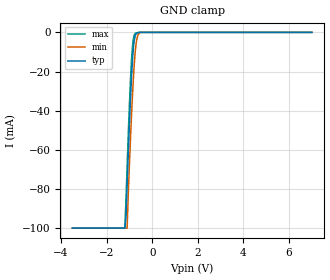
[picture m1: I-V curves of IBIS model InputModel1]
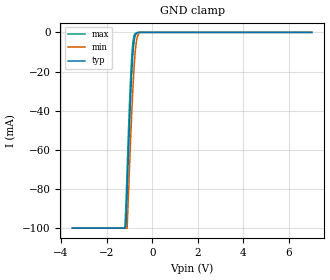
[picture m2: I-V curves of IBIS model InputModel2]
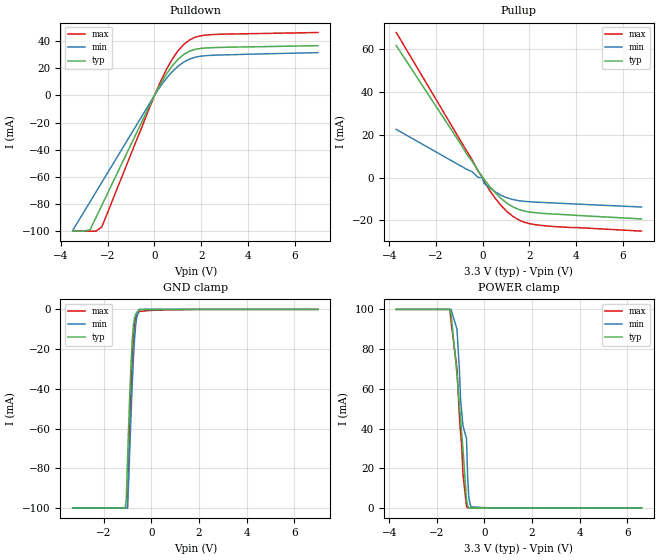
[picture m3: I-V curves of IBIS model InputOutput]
[IBIS Ver]   2.1
[File name]   pa016s33.ibs   | pa= PSOP, f016s3= abbr chip name, 3= 3.3V Vcc
[File Rev]   2.00
[Date]   18-April-1996
[Source]   File generated from lab measurements at Intel Corporation
[Notes]   Rev 2.00 All data was replaced by actual measurements
   performed in a lab.
[Disclaimer] INTEL DEVELOPER'S SOFTWARE LICENSE AGREEMENT
| BY USING THIS SOFTWARE, YOU ARE AGREEING TO BE BOUND
| BY THE TERMS OF THIS AGREEMENT.  DO NOT USE THE SOFTWARE
| UNTIL YOU HAVE CAREFULLY READ AND AGREED TO THE FOLLOWING
| TERMS AND CONDITIONS.  IF YOU DO NOT AGREE TO THE TERMS
| OF THIS AGREEMENT, PROMPTLY RETURN THE SOFTWARE PACKAGE
| AND ANY ACCOMPANYING ITEMS.
| IF YOU USE THIS SOFTWARE, YOU WILL BE BOUND BY THE TERMS
| OF THIS AGREEMENT
| LICENSE: Intel Corporation ("Intel") grants you the non-exclusive right
| to use the enclosed software program ("Software").  You will not use,
| copy, modify, rent, sell or transfer the Software or any portion
| thereof, except as provided in this Agreement.
| System OEM Developers may:
| 1.   Copy the Software for support, backup or archival purposes;
| 2.   Install, use, or distribute Intel owned Software in object code
|   only;
| 3.   Modify and/or use Software source code that Intel directly makes
|   available to you as an OEM Developer;
| 4.   Install, use, modify, distribute, and/or make or have made
|   derivatives ("Derivatives") of Intel owned Software under the
|   terms and conditions in this Agreement, ONLY if you are a System
|   OEM Developer and NOT an end-user.
| RESTRICTIONS:
| YOU WILL NOT:
| 1.   Copy the Software, in whole or in part, except as provided for
|   in this Agreement;
| 2.   Decompile or reverse engineer any Software provided in object
|   code format;
| 3.   Distribute any Software or Derivative code to any end-users,
|   unless approved by Intel in a prior writing.
| TRANSFER: You may transfer the Software to another OEM
| Developer if the receiving party agrees to the terms of this
| Agreement at the sole risk of any receiving party.
| OWNERSHIP AND COPYRIGHT OF SOFTWARE:
| Title to the Software and all copies thereof remain with Intel
| or its vendors.  The Software is copyrighted and is protected by
| United States and international copyright laws.  You will not
| remove the copyright notice from the Software.  You agree to
| prevent any unauthorized copying of the Software.
| DERIVATIVE WORK: OEM Developers that make or have made
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[Copyright]   Copyright 1996, Intel Corporation, All Rights Reserved
[Component]   PA28F016S3   | 44-lead PSOP package, 28F016S3
[Manufacturer]  Intel   | Flash File (tm)
|   | operating in 3V Vcc range
[Package]
|The following values apply for the leadframe.
|Variable   typ   min   max
R_pkg   145m   144m   147m
L_pkg   5.25nH   2.00nH   8.50nH
C_pkg   1.09pF   0.68pF   1.50pF
|*****************************Pin Definitions**********************************
[Pin]   signal_name   model_name   R_pin   L_pin   C_pin
  1   VPP   POWER
  2   RP#   InputModel1
  3   A11   InputModel1
  4   A10   InputModel1
  5   A09   InputModel1
  6   A08   InputModel1
  7   A07   InputModel1
  8   A06   InputModel1
  9   A05   InputModel1
 10   A04   InputModel1
 11   NC   InputModel2
 12   NC   InputModel2
 13   A03   InputModel1
 14   A02   InputModel1
 15   A01   InputModel1
 16   A00   InputModel1
 17   DQ0   InputOutput
 18   DQ1   InputOutput
 19   DQ2   InputOutput
 20   DQ3   InputOutput
 21   GND   GND
 22   GND   GND
 23   VCC   POWER
 24   DQ4   InputOutput
 25   DQ5   InputOutput
 26   DQ6   InputOutput
 27   DQ7   InputOutput
 28   RY/BY#   RYBYOutput
 29   OE#   InputModel2
 30   WE#   InputModel2
 31   NC   InputModel2
 32   NC   InputModel2
 33   NC   InputModel2
 34   A20   InputModel1
 35   A19   InputModel1
 36   A18   InputModel1
 37   A17   InputModel1
 38   A16   InputModel1
 39   A15   InputModel1
 40   A14   InputModel1
 41   A13   InputModel1
 42   A12   InputModel1
 43   CE#   InputModel1
 44   VCC   POWER
| Models and submodels in the file (4): InputModel1 (Input), InputModel2 (Input), InputOutput (I/O), RYBYOutput (Output)
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|**************************Input Model 1***************************************
[Model]   InputModel1
Model_type   Input
|   For A[0:20], CE# & RP#.
Vinl = 0.8V
Vinh = 2.0V
| Variable   typ   min   max
C_comp   5.61p   NA   7.6p
[Voltage Range]   3.3V   3.0V   3.6V
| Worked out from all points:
|   GND clamp passes 1 mA (typ) near -0.72 V on its own axis
[GND_clamp]
|Voltage I(typ)   I(min)   I(max)
-3.5V     -100mA     -100mA     -100mA
-1.2V     -100mA     -100mA     -100mA
-1.15V    -94.11mA   -100mA     -85.1mA
-1.1V     -77.66mA   -100mA     -68.19mA
-1.05V    -61.97mA   -82.63mA   -51.98mA
-950mV    -33.19mA   -53.62mA   -23.41mA
-900mV    -21.06mA   -40.46mA   -12.46mA
-850mV    -11.56mA   -28.75mA   -5.176mA
-750mV    -1.792mA   -10.47mA   -570.5uA
-650mV    -272.3uA   -2.213mA   -177.9uA
-500mV    0A         0A         0A
7V        0A         0A         0A
[POWER_clamp]
| Input buffer circuits of this product do not intrinsically
| require a [POWER_clamp] definition.  This zero current
| [POWER_clamp] is provided for compatibility with some ibis
| parsers.
|Voltage  I(typ)   I(min)   I(max)
-3.3V     0A         0A         0A
0V        0A         0A         0A
3.3V      0A         0A         0A
7V        0A         0A         0A
|**********************Input Model 2************************************
[Model]   InputModel2
Model_type   Input
|   For OE#, WE#, NC Pins
Vinl = 0.8V
Vinh = 2.0V
| Variable   typ   min   max
C_comp   5.61p   NA   7.6p
[Voltage Range]   3.3V   3.0V   3.6V
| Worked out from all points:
|   GND clamp passes 1 mA (typ) near -0.72 V on its own axis
[GND_clamp]
|Voltage I(typ)   I(min)   I(max)
-3.5V     -100mA     -100mA     -100mA
-1.2V     -100mA     -100mA     -100mA
-1.15V    -98.73mA   -100mA     -87.31mA
-1.1V     -81.6mA    -100mA     -69.85mA
-1V       -48.92mA   -70.34mA   -37.6mA
-900mV    -21.49mA   -41.83mA   -12.54mA
-850mV    -11.57mA   -29.48mA   -5.193mA
-800mV    -4.944mA   -18.71mA   -1.661mA
-750mV    -1.742mA   -10.48mA   -567.1uA
-650mV    -263.2uA   -2.181mA   0A
-550mV    0A         0A         0A
7V        0A         0A         0A
[POWER_clamp]
| Input buffer circuits of this product do not intrinsically
| require a [POWER_clamp] definition.  This zero current
| [POWER_clamp] is provided for compatibility with some ibis
| parsers.
|Voltage  I(typ)   I(min)   I(max)
-3.3V     0A         0A         0A
0V        0A         0A         0A
3.3V      0A         0A         0A
7V        0A         0A         0A
|**************************Input Output Model*********************************
[Model]   InputOutput
Model_type   I/O
|   for DQ[0:7]
Vinl = 0.8V
Vinh = 2.0V
| Variable   typ   min   max
C_comp   9.61p   NA   11.6p
[Voltage Range]   3.3V   3.0V   3.6V
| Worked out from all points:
|   slope of the pulldown table from 0 to 0.495 V, typ, clamps not added: 32.6 ohm
|   slope of the pullup table from 0 to 0.495 V, typ, clamps not added: 75.1 ohm
|   GND clamp passes 1 mA (typ) near -0.57 V on its own axis
|   POWER clamp passes 1 mA (typ) near -0.69 V on its own axis
[Pulldown]
| [Pullup] and [Pulldown] IV curves include only the current through
| the channels of output driver transistors when outputs are enabled
| with OE# = VIL.  Although the output driver transistors have np and
| pn diodes inherently created by CMOS IC fabrication between the
| drain and bulk of n-channel and p-channel CMOS transistors,
| the current through these junction diodes is not included in
| [Pullup] or [Pulldown].  Instead that drain/bulk diode current is
| included in the [POWER_clamp] or [GND_clamp] sections, which are
| not dependent on the state of OE# or output data value.
|Voltage  I(typ)   I(min)   I(max)
-3.5V     -100mA     -99.49mA   -100mA
-3V       -100mA     -85.29mA   -100mA
-2.75V    -98.83mA   -78.19mA   -100mA
-2.5V     -89.85mA   -71.09mA   -100mA
-2.25V    -80.88mA   -63.99mA   -96.85mA
0V        0A         0A         -208uA
250mV     8.097mA    6.516mA    9.821mA
750mV     21.46mA    17.25mA    26.36mA
1.25V     30.06mA    24.48mA    37.45mA
1.75V     33.91mA    28.15mA    42.88mA
2.25V     34.96mA    29.33mA    44.52mA
7V        36.6mA     31.5mA     46.3mA
[GND_clamp]
| [POWER_clamp] and [GND_clamp] IV curves describe ESD protection
| circuits PLUS some np and pn diodes which exist between the
| drain and bulk of n-channel and p-channel CMOS transistors.
| These drain/bulk diodes are inherent in CMOS IC fabrication,
| and are visible on the node of the I/O pin at all times.
| Even the drain/bulk diodes of output driver [Pullup] and [Powerdown]
| transistors are included in [POWER_clamp] or [GND_clamp], because
| these diodes contribute to I/O pin current even when the
| chip outputs are tristated by OE# = VIH.
| For example, when V forced on the I/O pin is large, we are
| forward biasing the pn diode at the drain/bulk interface in the
| p-channel pullup transistor.  Similarly, when V forced on the
| I/O pin is sufficiently negative with respect to the substrate
| ground, we are forward biasing the np diode at the drain/bulk
| interface in the n-channel pulldown transistor.  The effects
| of these diodes are included in [POWER_clamp] or [GND_clamp].
|Voltage  I(typ)   I(min)   I(max)
-3.3V     -100mA     -100mA     -100mA
-1.1V     -100mA     -100mA     -100mA
-1.05V    -96.11mA   -100mA     -100mA
-1V       -76.9mA    -100mA     -100mA
-950mV    -58.72mA   -86.94mA   -79.78mA
-850mV    -27.42mA   -53.11mA   -42.39mA
-800mV    -15.61mA   -37.97mA   -26.73mA
-750mV    -7.975mA   -24.86mA   -14.87mA
-700mV    -4.075mA   -14.58mA   -7.622mA
-650mV    -2.344mA   -7.543mA   -4.311mA
-500mV    0A         -88.2uA    -1.017mA
7V        0A         0A         0A
[Pullup]
| (Voltages for [Pullup] and [POWER_clamp] are specified with
| negative respect to Vcc.  Reference the IBIS documentation
| for more information regarding Vtable = Vcc - Voutput.
| This method keeps -Vds constant for the values in all three
| columns across a line of the table.
| [Pullup] and [Pulldown] IV curves include only the current through
| the channels of output driver transistors when outputs are enabled
| with OE# = VIL.  Although the output driver transistors have np and
| pn diodes inherently created by CMOS IC fabrication between the
| drain and bulk of n-channel and p-channel CMOS transistors,
| the current through these junction diodes is not included in
| [Pullup] or [Pulldown].  Instead that drain/bulk diode current is
| included in the [POWER_clamp] or [GND_clamp] sections, which are
| not dependent on the state of OE# or output data value.
|Voltage  I(typ)   I(min)   I(max)
-3.7V     61.75mA    22.54mA    67.88mA
-700mV    11.29mA    3.94mA     12.68mA
-450mV    7.529mA    2.716mA    8.241mA
-200mV    3.249mA    65.93uA    3.093mA
0V        0A         0A         0A
50mV      -663uA     -2.583mA   -1.683mA
300mV     -4.172mA   -4.875mA   -6.038mA
800mV     -9.924mA   -8.356mA   -13.25mA
1.05V     -12.08mA   -9.528mA   -16.04mA
1.55V     -14.96mA   -10.84mA   -19.88mA
2.3V      -16.53mA   -11.53mA   -22.15mA
6.8V      -19.38mA   -13.8mA    -25.08mA
[POWER_clamp]
| (Voltages for [Pullup] and [POWER_clamp] are specified with
| negative respect to Vcc.  Reference the IBIS documentation
| for more information regarding Vtable = Vcc - Voutput.
| This method keeps -Vds constant for the values in all three
| columns across a line of the table.
| [POWER_clamp] and [GND_clamp] IV curves describe ESD protection
| circuits PLUS some np and pn diodes which exist between the
| drain and bulk of n-channel and p-channel CMOS transistors.
| These drain/bulk diodes are inherent in CMOS IC fabrication,
| and are visible on the node of the I/O pin at all times.
| Even the drain/bulk diodes of output driver [Pullup] and [Powerdown]
| transistors are included in [POWER_clamp] or [GND_clamp], because
| these diodes contribute to I/O pin current even when the
| chip outputs are tristated by OE# = VIH.
| For example, when V forced on the I/O pin is large, we are
| forward biasing the pn diode at the drain/bulk interface in the
| p-channel pullup transistor.  Similarly, when V forced on the
| I/O pin is sufficiently negative with respect to the substrate
| ground, we are forward biasing the np diode at the drain/bulk
| interface in the n-channel pulldown transistor.  The effects
| of these diodes are included in [POWER_clamp] or [GND_clamp].
|Voltage  I(typ)   I(min)   I(max)
-3.7V     100mA      100mA      100mA
-1.45V    100mA      100mA      100mA
-1.4V     97.9mA     100mA      94.01mA
-1.15V    67.32mA    90mA       70mA
-1V       44.92mA    54.99mA    38mA
-950mV    37mA       48.19mA    31.04mA
-900mV    29.87mA    41.44mA    17.3mA
-750mV    3.994mA    35mA       792.4uA
-700mV    1.105mA    15mA       0A
-650mV    199.3uA    5.012mA    0A
-550mV    0A         539.7uA    0A
6.6V      0A         0A         0A
[Ramp]
| The DQ Ramp information is not provided at this time for the
| device but will be available in the future.  The table below
| is for the compatibility with some IBIS parsers.
| Variable   typ   min   max
 dV/dt_r   0V/0ns   0V/0ns   0V/0ns
 dV/dt_f   0V/0ns   0V/0ns   0V/0ns
